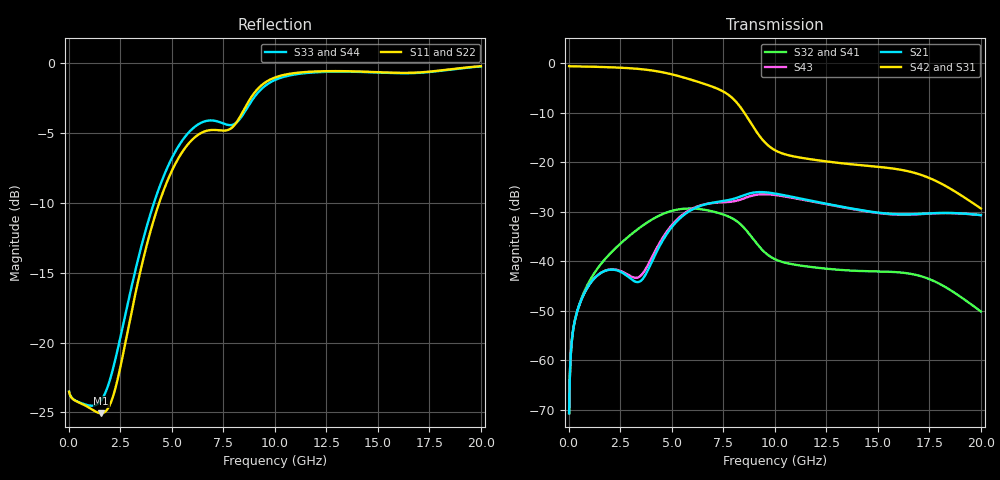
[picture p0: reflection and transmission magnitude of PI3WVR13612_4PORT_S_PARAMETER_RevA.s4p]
! NPort=4 DATA=800 NOISE=0 GROUPDELAY=0 COMPLEX_DATAFORMAT=POLAR
! NumOfBlock=1 NumOfParam=0
! .MODEL Smodel S TSTONEFILE=PI3WVR13612_4PORT_S_PARAMETER_RevA.s4p TYPE=S
!  -- The above .MODEL line can be used for the S element in the netlist.
! PORT DEFINITION
! PORT1 = INPUT+
! PORT2 = INPUT-
! PORT3 = OUTPUT+
! PORT4 = OUTPUT-
# Hz S MA R  50
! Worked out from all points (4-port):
!   800 points, 25 MHz to 20 GHz, reference 50 ohm
!   strongest paths, dB at 25 MHz, 5.025 GHz, 10.03 GHz, 15.03 GHz, 20 GHz:
!     S42: -0.6, -2.3, -17.6, -20.9, -29.3
!     S31: -0.6, -2.3, -17.7, -21.0, -29.4
!     S21: -70.6, -33.0, -26.3, -30.2, -30.7
!     S43: -70.6, -32.6, -26.6, -30.3, -30.7
!     S32: -70.7, -29.8, -39.6, -42.1, -50.1
!     S41: -70.7, -29.8, -39.6, -42.1, -50.1
!   lowest |S11| = -25.1 dB at 1.575 GHz (marker M1), VSWR 1.12, Z = 55.2 - j2.7 ohm
!   |S11| at or under -10 dB: start of sweep to 4.396 GHz
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2.5e7  0.0667 -2.6  0.0002936 86.0  0.9298 -0.7  0.0002922 85.9
       0.0002936 86.0  0.06672 -2.6  0.0002922 85.9  0.9298 -0.7
       0.9298 -0.7  0.0002922 85.9  0.06674 -2.4  0.0002936 86.0
       0.0002922 85.9  0.9298 -0.7  0.0002936 86.0  0.06672 -2.4
3.75e8  0.06169 -12.5  0.002901 62.6  0.9245 -9.0  0.002916 61.9
        0.0029 62.6  0.06173 -12.4  0.002916 61.9  0.9244 -9.0
        0.9244 -9.0  0.002916 61.9  0.06172 -9.0  0.002899 62.8
        0.002916 61.9  0.9245 -9.0  0.002899 62.8  0.06168 -9.1
1.575e9  0.05585 -25.9  0.00765 48.3  0.9129 -37.5  0.009414 44.5
         0.007647 48.3  0.05611 -25.4  0.009417 44.6  0.9129 -37.5
         0.9128 -37.5  0.009417 44.6  0.06204 -11.8  0.007657 49.4
         0.009414 44.5  0.9129 -37.5  0.00766 49.4  0.06189 -12.0
3.75e9  0.2171 -10.9  0.007432 82.8  0.8569 -92.1  0.02411 -6.2
        0.007435 82.9  0.2181 -11.0  0.02412 -6.2  0.8569 -92.1
        0.8567 -92.1  0.02412 -6.2  0.2537 -11.1  0.008422 82.0
        0.02411 -6.2  0.8571 -92.0  0.008419 81.9  0.2532 -11.1
6.125e9  0.5421 -59.5  0.03427 62.4  0.6609 -156.4  0.03394 -87.9
         0.03429 62.4  0.5431 -59.6  0.03395 -87.9  0.6609 -156.5
         0.6607 -156.5  0.03395 -87.9  0.5912 -61.7  0.03494 58.2
         0.03394 -87.9  0.6611 -156.4  0.03492 58.2  0.5907 -61.7
8.2e9  0.621 -75.6  0.04393 31.9  0.3893 136.4  0.02501 -160.9
       0.04393 31.9  0.6209 -75.7  0.025 -160.9  0.3894 136.3
       0.3891 136.3  0.025 -160.9  0.617 -81.1  0.04103 28.7
       0.025 -160.9  0.3896 136.4  0.04104 28.8  0.6167 -81.1
2e10  0.9733 -138.8  0.02922 -44.4  0.0341 1.3  0.003112 16.3
      0.02922 -44.4  0.9732 -138.8  0.003113 16.3  0.03405 0.9
      0.03406 1.1  0.003113 16.3  0.9714 -138.8  0.02919 -44.2
      0.003112 16.3  0.0341 1.1  0.02919 -44.1  0.9716 -138.8
